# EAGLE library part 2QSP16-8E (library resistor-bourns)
BOURNS RESISTOR NETWORK
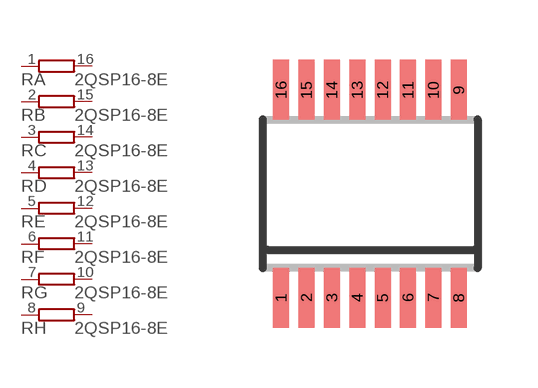
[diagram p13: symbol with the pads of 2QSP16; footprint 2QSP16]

Designator prefix R; gates A=R1NV B=R1NV C=R1NV D=R1NV E=R1NV F=R1NV G=R1NV H=R1NV

## 2QSP16-8E (OC_FARNELL: unknown; OC_NEWARK: unknown)  [2QSP16]
1  A:1  pas
2  B:1  pas
3  C:1  pas
4  D:1  pas
5  E:1  pas
6  F:1  pas
7  G:1  pas
8  H:1  pas
9  H:2  pas
10  G:2  pas
11  F:2  pas
12  E:2  pas
13  D:2  pas
14  C:2  pas
15  B:2  pas
16  A:2  pas

## Footprint 2QSP16 (pad centres in mm)
BOURNS RESISTOR NETWORK
smd 0.4 x 1.5: 1 -2.223,-2.6; 2 -1.588,-2.6; 3 -0.953,-2.6; 4 -0.318,-2.6; 5 0.318,-2.6; 6 0.953,-2.6; 7 1.588,-2.6; 8 2.223,-2.6; 9 2.223,2.6; 10 1.588,2.6; 11 0.953,2.6; 12 0.318,2.6; 13 -0.318,2.6; 14 -0.953,2.6; 15 -1.588,2.6; 16 -2.223,2.6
